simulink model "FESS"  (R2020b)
settings: Solver=VariableStepAuto  StartTime=0.0  StopTime=30  RelTol=1e-3
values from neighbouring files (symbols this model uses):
  C = 0    [FESS.m]
  F = 1    [FESS.m]
  f_el = 50    [FESS.m]
  P_load = 1500    [FESS.m]
  t_step = 5    [FESS.m]
undefined symbols (not defined in the file or in its folder): DCmot, DG
libraries: pid_lib x4, simulink x2

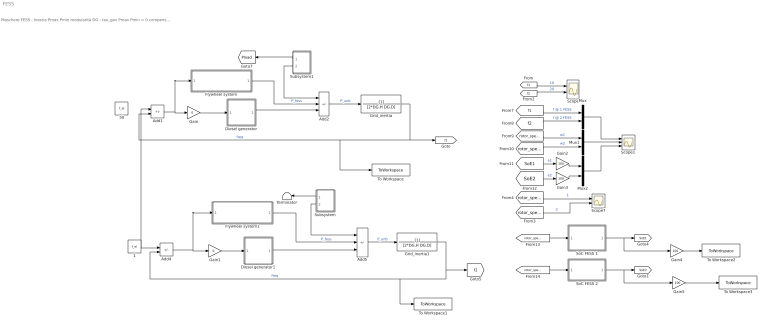
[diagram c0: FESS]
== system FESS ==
  note: Maschere FESS : Inerzia Pmax Pmin modularità DG : tau_gov Pmax Pmin = 0 compensazione FESS [0-1] Load : impulsi [0-1] step [0-1] Pstep Ptrain t/duty pulses
  1 : Constant  Value=f_el
  50 : Constant  Value=f_el
  Add1 : Sum  Inputs=+-
  Add2 : Sum  Inputs=-++
  Add4 : Sum  Inputs=+-
  Add5 : Sum  Inputs=-++
  Diesel generator : Subsystem  mask{s=[DG.tau_gov 1], W=4e5, O=-0.5, Gain=0}
      mask prompts: s "Tau_DG"; W "Upper limit P"; O "Lower limit P"; Gain "compensation"
  Diesel generator1 : Subsystem  mask{s=[DG.tau_gov 1], W=4e5, O=-0.5, Gain=0}
      mask prompts: s "Tau_DG"; W "Upper limit P"; O "Lower limit P"; Gain "compensation"
  Flywheel system : Subsystem  mask{J=20, Plim=DCmot.Pmax, Plim_neg=-DCmot.Pmax, Gain=1}
      mask prompts: J "Inerzia [kg*m^2]"; Plim "power limitation pos"; Plim_neg "power limitation neg"; Gain "Mod"
  Flywheel system1 : Subsystem  mask{J=20, Gain=1}
      mask prompts: J "Inerzia [kg*m^2]"; Gain "Mod"
  Gain : Gain  Gain=0
  Gain1 : Gain  Gain=0
  Gain{2..5} (4 alike) : Gain  Gain=100
  Grid_inertia : TransferFcn  Denominator=[2*DG.H DG.D]
  Grid_inertia1 : TransferFcn  Denominator=[2*DG.H DG.D]
  Mux : Mux  Inputs=2
  Mux1 : Mux  Inputs=2
  Mux2 : Mux  Inputs=2
  Scope : Scope  NumInputPorts=2
  Scope1 : Scope  NumInputPorts=3
  Scope7 : Scope  NumInputPorts=2
  SoC FESS 1 : Subsystem
  SoC FESS 2 : Subsystem
  Subsystem : Subsystem  mask{Gain=0, G=1, After=P_load, Amplitude=P_load, Period=3, PulseWidth=50}
      mask prompts: Gain "train"; G "step"; After "Pstep"; Amplitude "Puls amp"; Period "pulse durat"; PulseWidth "duty cycle"
  Subsystem1 : Subsystem  mask{Gain=1, G=0, After=P_load, Amplitude=P_load*2, Period=3, PulseWidth=50}
      mask prompts: Gain "train"; G "step"; After "Pstep"; Amplitude "Puls amp"; Period "pulse durat"; PulseWidth "duty cycle"
  Terminator : Terminator
  To Workspace : ToWorkspace  VariableName=f1  SaveFormat=Timeseries  SampleTime=-1
  To Workspace1 : ToWorkspace  VariableName=f2  SaveFormat=Timeseries  SampleTime=-1
  To Workspace2 : ToWorkspace  VariableName=Soe1  SaveFormat=Timeseries  SampleTime=-1
  To Workspace3 : ToWorkspace  VariableName=Soe2  SaveFormat=Timeseries  SampleTime=-1
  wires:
  Add1/1 -> Flywheel system/1(e_f), Gain/1
  Add2/1 -> Grid_inertia/1  "P_unb"
  50/1 -> Add1/1
  Grid_inertia/1 -> To Workspace/1, Add1/2, [f1]  "freq"
  Grid_inertia1/1 -> To Workspace1/1, Add4/2, [f2]  "freq"
  1/1 -> Add4/1
  Add5/1 -> Grid_inertia1/1  "P_unb"
  Add4/1 -> Flywheel system1/1(e_f), Gain1/1
  [f1] -> Scope/1  "10"
  Diesel generator/1(P_out) -> Add2/3
  Flywheel system1/1(P_FESS) -> Add5/2  "P_fess"
  Diesel generator1/1(P_out) -> Add5/3
  Subsystem/2(Pl) -> Add5/1
  Subsystem1/1(load) -> [Pload]
  Flywheel system/1(P_FESS) -> Add2/2  "P_fess"
  Subsystem1/2(Pl) -> Add2/1
  Subsystem/1(load) -> Terminator/1
  [f2] -> Scope/2  "20"
  Gain/1 -> Diesel generator/1(e_f)
  Gain1/1 -> Diesel generator1/1(e_f)
  [rotor_speed2] -> Scope7/2  "2"
  [rotor_speed2] -> SoC FESS 2/1(speed)
  SoC FESS 1/1(SoE) -> Gain4/1, [SoE1]
  [rotor_speed1] -> Scope7/1  "1"
  [rotor_speed1] -> SoC FESS 1/1(speed1)
  SoC FESS 2/1(SoE) -> Gain5/1, [SoE2]
  [rotor_speed1] -> Mux1/1  "w1"
  [SoE2] -> Gain3/1  "e2"
  [f1] -> Mux/1  "f @ 1 FESS"
  Mux/1 -> Scope1/1
  [f2] -> Mux/2  "f @ 2 FESS"
  [SoE1] -> Gain2/1  "e1"
  Mux1/1 -> Scope1/2
  [rotor_speed2] -> Mux1/2  "w2"
  Mux2/1 -> Scope1/3
  Gain2/1 -> Mux2/1
  Gain3/1 -> Mux2/2
  Gain4/1 -> To Workspace2/1
  Gain5/1 -> To Workspace3/1

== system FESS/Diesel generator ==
  note: aggiungo la Pload
  e_f : Inport
  Add : Sum
  Governor : TransferFcn  Denominator=s
  PI_DG : Subsystem
  Pload_compensation : Gain  Gain=Gain
  Saturation : Saturate  UpperLimit=W  LowerLimit=O
  P_out : Outport
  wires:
  Saturation/1 -> Governor/1
  Pload_compensation/1 -> Add/1
  Add/1 -> Saturation/1
  PI_DG/1(P_ref) -> Add/2
  e_f/1 -> PI_DG/1(e_f)
  [Pload] -> Pload_compensation/1
  Governor/1 -> P_out/1

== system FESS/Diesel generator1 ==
  note: aggiungo la Pload
  e_f : Inport
  Add : Sum
  Governor : TransferFcn  Denominator=s
  PI_DG : Subsystem
  Pload_compensation : Gain  Gain=Gain
  Saturation : Saturate  UpperLimit=W  LowerLimit=O
  P_out : Outport
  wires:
  Governor/1 -> P_out/1
  [Pload] -> Pload_compensation/1
  e_f/1 -> PI_DG/1(e_f)
  PI_DG/1(P_ref) -> Add/2
  Add/1 -> Saturation/1
  Pload_compensation/1 -> Add/1
  Saturation/1 -> Governor/1

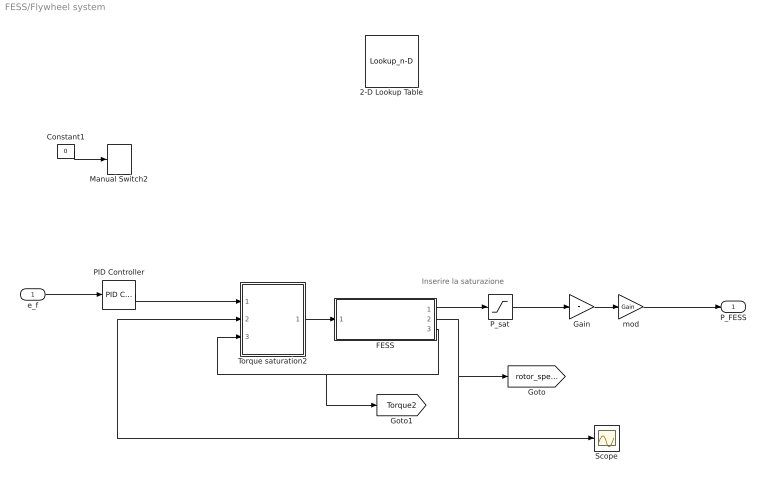
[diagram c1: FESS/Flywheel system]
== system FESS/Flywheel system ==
  note: Inserire la saturazione
  e_f : Inport
  2-D Lookup Table : Lookup_n-D  Commented=on  BreakpointsForDimension1=[1:3]  BreakpointsForDimension2=[1:3]  InternalRulePriority=Speed  RndMeth=Simplest
  Constant1 : Constant  Commented=on  Value=0
  FESS : Subsystem
  Gain : Gain  Gain=F
  Manual Switch2 : ManualSwitch  Commented=on  CurrentSetting=0
  PID Controller : pid_lib/PID Controller  Controller=PID  Form=Parallel  TimeDomain=Continuous-time  UseExternalTs=off  SampleTime=-1  IntegratorMethod=Forward Euler  FilterMethod=Forward Euler  ControllerParametersSource=internal  P=50*DCmot.Kt  I=100  D=0  UseFilter=on  N=100  TunerSelectOption=Transfer Function Based (PID Tuner App)  InitialConditionSource=internal  InitialConditionForIntegrator=0  InitialConditionForFilter=0  DifferentiatorICPrevScaledInput=0  ExternalReset=none  TrackingMode=off  Kt=1  LimitOutput=off  SatLimitsSource=internal  UpperSaturationLimit=inf  LowerSaturationLimit=-inf  LinearizeAsGain=on  AntiWindupMode=none  Kb=1  POutMin=[]  POutMax=[]  IOutMin=[]  IOutMax=[]  DOutMin=[]  DOutMax=[]  NOutMin=[]  NOutMax=[]  SumOutMin=[]  SumOutMax=[]  SaturationOutMin=[]  SaturationOutMax=[]  PParamMin=[]  PParamMax=[]  IParamMin=[]  IParamMax=[]  DParamMin=[]  DParamMax=[]  NParamMin=[]  NParamMax=[]  KbParamMin=[]  KbParamMax=[]  KtParamMin=[]  KtParamMax=[]  KbOutMin=[]  KbOutMax=[]  KtOutMin=[]  KtOutMax=[]  IntegratorOutMin=[]  IntegratorOutMax=[]  FilterOutMin=[]  FilterOutMax=[]  SumI1OutMin=[]  SumI1OutMax=[]  SumI2OutMin=[]  SumI2OutMax=[]  SumI3OutMin=[]  SumI3OutMax=[]  SumI4OutMin=[]  SumI4OutMax=[]  SumDOutMin=[]  SumDOutMax=[]  DifferentiatorOutMin=[]  DifferentiatorOutMax=[]  FilterDiffOutCoefMin=[]  FilterDiffOutCoefMax=[]  ReciprocalOutMin=[]  ReciprocalOutMax=[]  SumDenOutMin=[]  SumDenOutMax=[]  SumNumOutMin=[]  SumNumOutMax=[]  DivideOutMin=[]  DivideOutMax=[]  UdiffTsProdOutMin=[]  UdiffTsProdOutMax=[]  NTsProdOutMin=[]  NTsProdOutMax=[]  UintegralTsProdOutMin=[]  UintegralTsProdOutMax=[]  UngainTsProdOutMin=[]  UngainTsProdOutMax=[]  IntegratorContinuousStateAttributes=''  IntegratorStateMustResolveToSignalObject=off  IntegratorRTWStateStorageClass=Auto  FilterContinuousStateAttributes=''  FilterStateMustResolveToSignalObject=off  FilterRTWStateStorageClass=Auto  ParallelPVariant=InternalParameters  IdealPVariant=Disabled  IVariant=InternalParameters  DVariant=InternalParameters  IntegratorVariant=Continuous  SatVariant=Disabled  AWVariant=Passthrough  PCopyVariant=Disabled  TRVariant=Disabled  FdbkBlocksVariant=Forward  IdealPFdbkVariant=Disabled  SatFdbkVariant=Disabled  DerivativeFilterVariant=ContFilter  NVariant=InternalParameters  NCopyVariant=Disabled  FilterICVariant=InternalICsFilter  IntegratorICVariant=InternalICs  ExternalResetVariant=Disabled  TRSumVariant=Passthrough  SumFdbkVariant=Disabled  SumVariant=Sum_PID  TsampFilterVariant=InternalTs  TsampNgainVariant=Passthrough  TsampIntegralVariant=Passthrough  ExternalSaturationOutDataTypeStr=Inherit: Same as second input
  P_sat : Saturate  UpperLimit=Plim  LowerLimit=Plim_neg
  Scope : Scope
  Torque saturation2 : Subsystem
  mod : Gain  Gain=Gain
  P_FESS : Outport
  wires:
  e_f/1 -> PID Controller/1
  Torque saturation2/1(ia*) -> FESS/1(ia_ref)
  PID Controller/1 -> Torque saturation2/1(T*)
  FESS/2(w_r) -> [rotor_speed1], Torque saturation2/2(speed), Scope/1
  FESS/3(Tm) -> [Torque2], Torque saturation2/3(Torque)
  Constant1/1 -> Manual Switch2/1
  FESS/1(P_FESS) -> P_sat/1
  Gain/1 -> mod/1
  mod/1 -> P_FESS/1
  P_sat/1 -> Gain/1

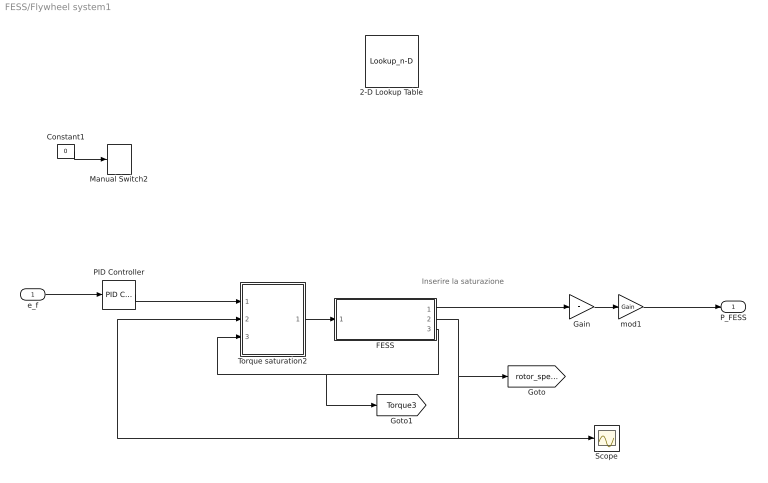
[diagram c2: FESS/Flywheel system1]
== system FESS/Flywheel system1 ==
  note: Inserire la saturazione
  e_f : Inport
  2-D Lookup Table : Lookup_n-D  Commented=on  BreakpointsForDimension1=[1:3]  BreakpointsForDimension2=[1:3]  InternalRulePriority=Speed  RndMeth=Simplest
  Constant1 : Constant  Commented=on  Value=0
  FESS : Subsystem
  Gain : Gain  Gain=F
  Manual Switch2 : ManualSwitch  Commented=on  CurrentSetting=0
  PID Controller : pid_lib/PID Controller  Controller=PID  Form=Parallel  TimeDomain=Continuous-time  UseExternalTs=off  SampleTime=-1  IntegratorMethod=Forward Euler  FilterMethod=Forward Euler  ControllerParametersSource=internal  P=50*DCmot.Kt  I=100  D=0  UseFilter=on  N=100  TunerSelectOption=Transfer Function Based (PID Tuner App)  InitialConditionSource=internal  InitialConditionForIntegrator=0  InitialConditionForFilter=0  DifferentiatorICPrevScaledInput=0  ExternalReset=none  TrackingMode=off  Kt=1  LimitOutput=off  SatLimitsSource=internal  UpperSaturationLimit=inf  LowerSaturationLimit=-inf  LinearizeAsGain=on  AntiWindupMode=none  Kb=1  POutMin=[]  POutMax=[]  IOutMin=[]  IOutMax=[]  DOutMin=[]  DOutMax=[]  NOutMin=[]  NOutMax=[]  SumOutMin=[]  SumOutMax=[]  SaturationOutMin=[]  SaturationOutMax=[]  PParamMin=[]  PParamMax=[]  IParamMin=[]  IParamMax=[]  DParamMin=[]  DParamMax=[]  NParamMin=[]  NParamMax=[]  KbParamMin=[]  KbParamMax=[]  KtParamMin=[]  KtParamMax=[]  KbOutMin=[]  KbOutMax=[]  KtOutMin=[]  KtOutMax=[]  IntegratorOutMin=[]  IntegratorOutMax=[]  FilterOutMin=[]  FilterOutMax=[]  SumI1OutMin=[]  SumI1OutMax=[]  SumI2OutMin=[]  SumI2OutMax=[]  SumI3OutMin=[]  SumI3OutMax=[]  SumI4OutMin=[]  SumI4OutMax=[]  SumDOutMin=[]  SumDOutMax=[]  DifferentiatorOutMin=[]  DifferentiatorOutMax=[]  FilterDiffOutCoefMin=[]  FilterDiffOutCoefMax=[]  ReciprocalOutMin=[]  ReciprocalOutMax=[]  SumDenOutMin=[]  SumDenOutMax=[]  SumNumOutMin=[]  SumNumOutMax=[]  DivideOutMin=[]  DivideOutMax=[]  UdiffTsProdOutMin=[]  UdiffTsProdOutMax=[]  NTsProdOutMin=[]  NTsProdOutMax=[]  UintegralTsProdOutMin=[]  UintegralTsProdOutMax=[]  UngainTsProdOutMin=[]  UngainTsProdOutMax=[]  IntegratorContinuousStateAttributes=''  IntegratorStateMustResolveToSignalObject=off  IntegratorRTWStateStorageClass=Auto  FilterContinuousStateAttributes=''  FilterStateMustResolveToSignalObject=off  FilterRTWStateStorageClass=Auto  ParallelPVariant=InternalParameters  IdealPVariant=Disabled  IVariant=InternalParameters  DVariant=InternalParameters  IntegratorVariant=Continuous  SatVariant=Disabled  AWVariant=Passthrough  PCopyVariant=Disabled  TRVariant=Disabled  FdbkBlocksVariant=Forward  IdealPFdbkVariant=Disabled  SatFdbkVariant=Disabled  DerivativeFilterVariant=ContFilter  NVariant=InternalParameters  NCopyVariant=Disabled  FilterICVariant=InternalICsFilter  IntegratorICVariant=InternalICs  ExternalResetVariant=Disabled  TRSumVariant=Passthrough  SumFdbkVariant=Disabled  SumVariant=Sum_PID  TsampFilterVariant=InternalTs  TsampNgainVariant=Passthrough  TsampIntegralVariant=Passthrough  ExternalSaturationOutDataTypeStr=Inherit: Same as second input
  Scope : Scope
  Torque saturation2 : Subsystem
  mod1 : Gain  Gain=Gain
  P_FESS : Outport
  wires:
  e_f/1 -> PID Controller/1
  Torque saturation2/1(ia*) -> FESS/1(ia_ref)
  PID Controller/1 -> Torque saturation2/1(T*)
  FESS/2(w_r) -> [rotor_speed2], Torque saturation2/2(speed), Scope/1
  FESS/3(Tm) -> [Torque3], Torque saturation2/3(Torque)
  Constant1/1 -> Manual Switch2/1
  FESS/1(P_FESS) -> Gain/1
  Gain/1 -> mod1/1
  mod1/1 -> P_FESS/1

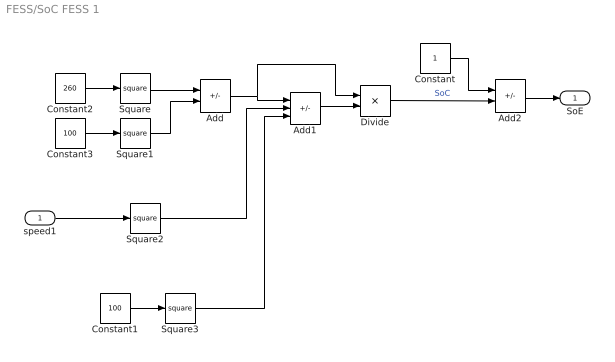
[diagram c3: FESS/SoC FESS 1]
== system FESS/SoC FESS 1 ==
  speed1 : Inport
  Add : Sum  Inputs=+-
  Add1 : Sum  Inputs=+-+
  Add2 : Sum  Inputs=+-
  Constant : Constant
  Constant1 : Constant  Value=100
  Constant2 : Constant  Value=260
  Constant3 : Constant  Value=100
  Divide : Product  Inputs=/*
  Square{,1..3} (4 alike) : Math  Operator=square
  SoE : Outport
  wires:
  Constant2/1 -> Square/1
  Divide/1 -> Add2/2  "SoC"
  Add1/1 -> Divide/2
  Add/1 -> Divide/1, Add1/1
  Constant3/1 -> Square1/1
  Square/1 -> Add/1
  Square1/1 -> Add/2
  Square2/1 -> Add1/2
  Square3/1 -> Add1/3
  Constant1/1 -> Square3/1
  Constant/1 -> Add2/1
  Add2/1 -> SoE/1
  speed1/1 -> Square2/1

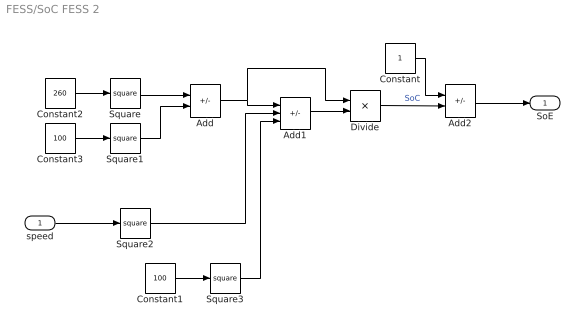
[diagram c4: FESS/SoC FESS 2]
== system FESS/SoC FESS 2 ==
  speed : Inport
  Add : Sum  Inputs=+-
  Add1 : Sum  Inputs=+-+
  Add2 : Sum  Inputs=+-
  Constant : Constant
  Constant1 : Constant  Value=100
  Constant2 : Constant  Value=260
  Constant3 : Constant  Value=100
  Divide : Product  Inputs=/*
  Square{,1..3} (4 alike) : Math  Operator=square
  SoE : Outport
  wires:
  Square2/1 -> Add1/2
  speed/1 -> Square2/1
  Square1/1 -> Add/2
  Square/1 -> Add/1
  Constant3/1 -> Square1/1
  Add/1 -> Add1/1, Divide/1
  Add1/1 -> Divide/2
  Divide/1 -> Add2/2  "SoC"
  Constant2/1 -> Square/1
  Constant1/1 -> Square3/1
  Square3/1 -> Add1/3
  Constant/1 -> Add2/1
  Add2/1 -> SoE/1

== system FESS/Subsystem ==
  Add : Sum
  P_load2 : Step  Time=t_step  After=After  SampleTime=0
  Positive Load1 : DiscretePulseGenerator  PulseType=Time based  Amplitude=Amplitude  Period=Period  PulseWidth=PulseWidth
  step : Gain  Gain=G
  train : Gain  Gain=Gain
  load : Outport
  Pl : Outport  Port=2
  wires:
  step/1 -> Add/1
  P_load2/1 -> step/1, load/1  "load"
  train/1 -> Add/2
  Positive Load1/1 -> train/1
  Add/1 -> Pl/1

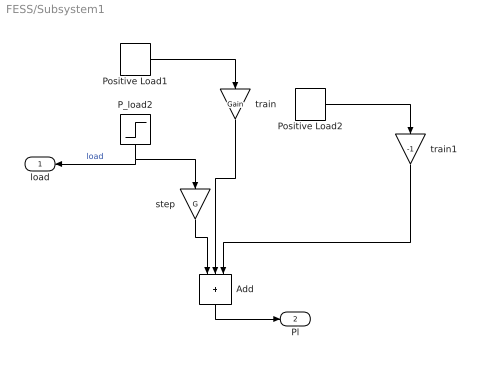
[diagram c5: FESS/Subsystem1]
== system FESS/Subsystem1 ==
  Add : Sum  Inputs=+++
  P_load2 : Step  Time=t_step  After=After  SampleTime=0
  Positive Load1 : DiscretePulseGenerator  PulseType=Time based  Amplitude=Amplitude  Period=Period  PulseWidth=PulseWidth
  Positive Load2 : DiscretePulseGenerator  PulseType=Time based  Amplitude=P_load  Period=3  PulseWidth=50  PhaseDelay=1.5
  step : Gain  Gain=G
  train : Gain  Gain=Gain
  train1 : Gain  Gain=-1
  load : Outport
  Pl : Outport  Port=2
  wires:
  step/1 -> Add/1
  P_load2/1 -> step/1, load/1  "load"
  train/1 -> Add/2
  Positive Load1/1 -> train/1
  Add/1 -> Pl/1
  Positive Load2/1 -> train1/1
  train1/1 -> Add/3

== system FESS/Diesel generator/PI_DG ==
  e_f : Inport
  Add : Sum
  Integrator : Integrator
  Ki,DG : Gain  Gain=DG.ki_dg
  Kp,DG : Gain  Gain=DG.kp_dg
  Manual Switch : ManualSwitch  CurrentSetting=0
  PID Controller : pid_lib/PID Controller  Controller=PID  Form=Parallel  TimeDomain=Continuous-time  UseExternalTs=off  SampleTime=-1  IntegratorMethod=Forward Euler  FilterMethod=Forward Euler  ControllerParametersSource=internal  P=DG.kp_dg  I=DG.ki_dg  D=0  UseFilter=on  N=100  TunerSelectOption=Transfer Function Based (PID Tuner App)  InitialConditionSource=internal  InitialConditionForIntegrator=0  InitialConditionForFilter=0  DifferentiatorICPrevScaledInput=0  ExternalReset=none  TrackingMode=off  Kt=1  LimitOutput=off  SatLimitsSource=internal  UpperSaturationLimit=inf  LowerSaturationLimit=-inf  LinearizeAsGain=on  AntiWindupMode=none  Kb=1  POutMin=[]  POutMax=[]  IOutMin=[]  IOutMax=[]  DOutMin=[]  DOutMax=[]  NOutMin=[]  NOutMax=[]  SumOutMin=[]  SumOutMax=[]  SaturationOutMin=[]  SaturationOutMax=[]  PParamMin=[]  PParamMax=[]  IParamMin=[]  IParamMax=[]  DParamMin=[]  DParamMax=[]  NParamMin=[]  NParamMax=[]  KbParamMin=[]  KbParamMax=[]  KtParamMin=[]  KtParamMax=[]  KbOutMin=[]  KbOutMax=[]  KtOutMin=[]  KtOutMax=[]  IntegratorOutMin=[]  IntegratorOutMax=[]  FilterOutMin=[]  FilterOutMax=[]  SumI1OutMin=[]  SumI1OutMax=[]  SumI2OutMin=[]  SumI2OutMax=[]  SumI3OutMin=[]  SumI3OutMax=[]  SumI4OutMin=[]  SumI4OutMax=[]  SumDOutMin=[]  SumDOutMax=[]  DifferentiatorOutMin=[]  DifferentiatorOutMax=[]  FilterDiffOutCoefMin=[]  FilterDiffOutCoefMax=[]  ReciprocalOutMin=[]  ReciprocalOutMax=[]  SumDenOutMin=[]  SumDenOutMax=[]  SumNumOutMin=[]  SumNumOutMax=[]  DivideOutMin=[]  DivideOutMax=[]  UdiffTsProdOutMin=[]  UdiffTsProdOutMax=[]  NTsProdOutMin=[]  NTsProdOutMax=[]  UintegralTsProdOutMin=[]  UintegralTsProdOutMax=[]  UngainTsProdOutMin=[]  UngainTsProdOutMax=[]  IntegratorContinuousStateAttributes=''  IntegratorStateMustResolveToSignalObject=off  IntegratorRTWStateStorageClass=Auto  FilterContinuousStateAttributes=''  FilterStateMustResolveToSignalObject=off  FilterRTWStateStorageClass=Auto  ParallelPVariant=InternalParameters  IdealPVariant=Disabled  IVariant=InternalParameters  DVariant=InternalParameters  IntegratorVariant=Continuous  SatVariant=Disabled  AWVariant=Passthrough  PCopyVariant=Disabled  TRVariant=Disabled  FdbkBlocksVariant=Forward  IdealPFdbkVariant=Disabled  SatFdbkVariant=Disabled  DerivativeFilterVariant=ContFilter  NVariant=InternalParameters  NCopyVariant=Disabled  FilterICVariant=InternalICsFilter  IntegratorICVariant=InternalICs  ExternalResetVariant=Disabled  TRSumVariant=Passthrough  SumFdbkVariant=Disabled  SumVariant=Sum_PID  TsampFilterVariant=InternalTs  TsampNgainVariant=Passthrough  TsampIntegralVariant=Passthrough  ExternalSaturationOutDataTypeStr=Inherit: Same as second input
  P_ref : Outport
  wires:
  Integrator/1 -> Add/2
  e_f/1 -> PID Controller/1, Ki,DG/1, Kp,DG/1
  Kp,DG/1 -> Add/1
  Ki,DG/1 -> Integrator/1
  Add/1 -> Manual Switch/2
  Manual Switch/1 -> P_ref/1
  PID Controller/1 -> Manual Switch/1

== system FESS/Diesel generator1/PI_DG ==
  e_f : Inport
  Add : Sum
  Integrator : Integrator
  Ki,DG : Gain  Gain=DG.ki_dg
  Kp,DG : Gain  Gain=DG.kp_dg
  Manual Switch : ManualSwitch  CurrentSetting=0
  PID Controller : pid_lib/PID Controller  Controller=PID  Form=Parallel  TimeDomain=Continuous-time  UseExternalTs=off  SampleTime=-1  IntegratorMethod=Forward Euler  FilterMethod=Forward Euler  ControllerParametersSource=internal  P=DG.kp_dg  I=DG.ki_dg  D=0  UseFilter=on  N=100  TunerSelectOption=Transfer Function Based (PID Tuner App)  InitialConditionSource=internal  InitialConditionForIntegrator=0  InitialConditionForFilter=0  DifferentiatorICPrevScaledInput=0  ExternalReset=none  TrackingMode=off  Kt=1  LimitOutput=off  SatLimitsSource=internal  UpperSaturationLimit=inf  LowerSaturationLimit=-inf  LinearizeAsGain=on  AntiWindupMode=none  Kb=1  POutMin=[]  POutMax=[]  IOutMin=[]  IOutMax=[]  DOutMin=[]  DOutMax=[]  NOutMin=[]  NOutMax=[]  SumOutMin=[]  SumOutMax=[]  SaturationOutMin=[]  SaturationOutMax=[]  PParamMin=[]  PParamMax=[]  IParamMin=[]  IParamMax=[]  DParamMin=[]  DParamMax=[]  NParamMin=[]  NParamMax=[]  KbParamMin=[]  KbParamMax=[]  KtParamMin=[]  KtParamMax=[]  KbOutMin=[]  KbOutMax=[]  KtOutMin=[]  KtOutMax=[]  IntegratorOutMin=[]  IntegratorOutMax=[]  FilterOutMin=[]  FilterOutMax=[]  SumI1OutMin=[]  SumI1OutMax=[]  SumI2OutMin=[]  SumI2OutMax=[]  SumI3OutMin=[]  SumI3OutMax=[]  SumI4OutMin=[]  SumI4OutMax=[]  SumDOutMin=[]  SumDOutMax=[]  DifferentiatorOutMin=[]  DifferentiatorOutMax=[]  FilterDiffOutCoefMin=[]  FilterDiffOutCoefMax=[]  ReciprocalOutMin=[]  ReciprocalOutMax=[]  SumDenOutMin=[]  SumDenOutMax=[]  SumNumOutMin=[]  SumNumOutMax=[]  DivideOutMin=[]  DivideOutMax=[]  UdiffTsProdOutMin=[]  UdiffTsProdOutMax=[]  NTsProdOutMin=[]  NTsProdOutMax=[]  UintegralTsProdOutMin=[]  UintegralTsProdOutMax=[]  UngainTsProdOutMin=[]  UngainTsProdOutMax=[]  IntegratorContinuousStateAttributes=''  IntegratorStateMustResolveToSignalObject=off  IntegratorRTWStateStorageClass=Auto  FilterContinuousStateAttributes=''  FilterStateMustResolveToSignalObject=off  FilterRTWStateStorageClass=Auto  ParallelPVariant=InternalParameters  IdealPVariant=Disabled  IVariant=InternalParameters  DVariant=InternalParameters  IntegratorVariant=Continuous  SatVariant=Disabled  AWVariant=Passthrough  PCopyVariant=Disabled  TRVariant=Disabled  FdbkBlocksVariant=Forward  IdealPFdbkVariant=Disabled  SatFdbkVariant=Disabled  DerivativeFilterVariant=ContFilter  NVariant=InternalParameters  NCopyVariant=Disabled  FilterICVariant=InternalICsFilter  IntegratorICVariant=InternalICs  ExternalResetVariant=Disabled  TRSumVariant=Passthrough  SumFdbkVariant=Disabled  SumVariant=Sum_PID  TsampFilterVariant=InternalTs  TsampNgainVariant=Passthrough  TsampIntegralVariant=Passthrough  ExternalSaturationOutDataTypeStr=Inherit: Same as second input
  P_ref : Outport
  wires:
  PID Controller/1 -> Manual Switch/1
  Manual Switch/1 -> P_ref/1
  Add/1 -> Manual Switch/2
  Ki,DG/1 -> Integrator/1
  Kp,DG/1 -> Add/1
  e_f/1 -> Kp,DG/1, Ki,DG/1, PID Controller/1
  Integrator/1 -> Add/2

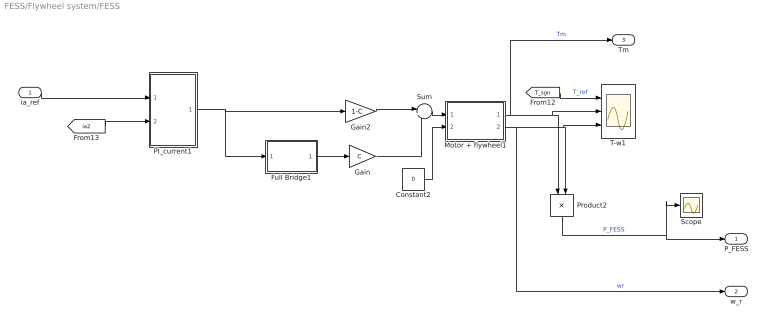
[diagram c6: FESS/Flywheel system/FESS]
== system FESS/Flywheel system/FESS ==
  ia_ref : Inport
  Constant2 : Constant  Value=0
  Full Bridge1 : Subsystem
  Gain : Gain  Gain=C
  Gain2 : Gain  Gain=1-C
  Motor + flywheel1 : Subsystem
  PI_current1 : Subsystem
  Product2 : Product
  Scope : Scope
  Sum : Sum  Inputs=|++
  T-w1 : Scope  NumInputPorts=3
  P_FESS : Outport
  w_r : Outport  Port=2
  Tm : Outport  Port=3
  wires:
  Motor + flywheel1/1(Tm) -> Tm/1, T-w1/2, Product2/1  "Tm"
  [ia2] -> PI_current1/2(ia_fbk)
  PI_current1/1(Va*) -> Gain2/1, Full Bridge1/1(Va_Ref)
  Constant2/1 -> Motor + flywheel1/2(Tr)
  Motor + flywheel1/2(wr) -> w_r/1, T-w1/3, Product2/2  "wr"
  [T_sgn] -> T-w1/1  "T_ref"
  ia_ref/1 -> PI_current1/1(ia*)
  Product2/1 -> Scope/1, P_FESS/1  "P_FESS"
  Full Bridge1/1(Va) -> Gain/1
  Gain2/1 -> Sum/1
  Sum/1 -> Motor + flywheel1/1(Va)
  Gain/1 -> Sum/2

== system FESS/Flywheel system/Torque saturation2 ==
  T* : Inport
  speed : Inport  Port=2
  Torque : Inport  Port=3
  Gain1 : Gain  Gain=1/DCmot.Kt
  Lookup with Linear Point-slope Interpolation : Lookup_n-D  NumberOfTableDimensions=1  BreakpointsForDimension1=[0,50,100,150,160,170,180,200,220,240,260]  Table=[0,0,0,1,1,1,1,1,1,1,0]  InternalRulePriority=Speed  RndMeth=Simplest
  MATLAB Function : MATLAB Function  Commented=on  TreatAsAtomicUnit=on
  Product2 : Product
  ia* : Outport
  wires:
  Lookup with Linear Point-slope Interpolation/1 -> Product2/2
  speed/1 -> Lookup with Linear Point-slope Interpolation/1
  Product2/1 -> Gain1/1
  T*/1 -> Product2/1
  Gain1/1 -> ia*/1
  Torque/1 -> MATLAB Function/2(T)

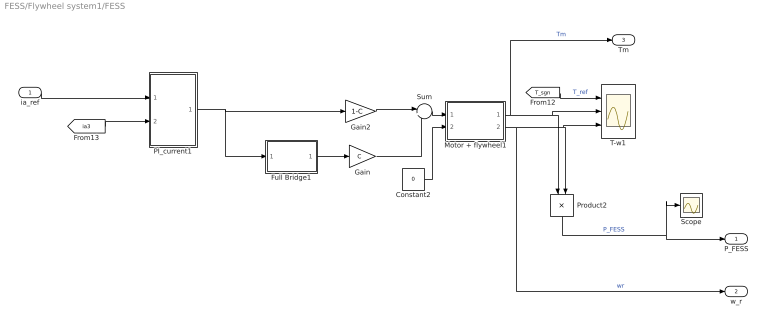
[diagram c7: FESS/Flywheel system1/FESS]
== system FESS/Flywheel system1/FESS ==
  ia_ref : Inport
  Constant2 : Constant  Value=0
  Full Bridge1 : Subsystem
  Gain : Gain  Gain=C
  Gain2 : Gain  Gain=1-C
  Motor + flywheel1 : Subsystem
  PI_current1 : Subsystem
  Product2 : Product
  Scope : Scope
  Sum : Sum  Inputs=|++
  T-w1 : Scope  NumInputPorts=3
  P_FESS : Outport
  w_r : Outport  Port=2
  Tm : Outport  Port=3
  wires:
  Motor + flywheel1/1(Tm) -> Tm/1, T-w1/2, Product2/1  "Tm"
  [ia3] -> PI_current1/2(ia_fbk)
  PI_current1/1(Va*) -> Gain2/1, Full Bridge1/1(Va_Ref)
  Constant2/1 -> Motor + flywheel1/2(Tr)
  Motor + flywheel1/2(wr) -> w_r/1, T-w1/3, Product2/2  "wr"
  [T_sgn] -> T-w1/1  "T_ref"
  ia_ref/1 -> PI_current1/1(ia*)
  Product2/1 -> Scope/1, P_FESS/1  "P_FESS"
  Full Bridge1/1(Va) -> Gain/1
  Gain2/1 -> Sum/1
  Sum/1 -> Motor + flywheel1/1(Va)
  Gain/1 -> Sum/2

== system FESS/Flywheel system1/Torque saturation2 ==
  T* : Inport
  speed : Inport  Port=2
  Torque : Inport  Port=3
  Gain1 : Gain  Gain=1/DCmot.Kt
  Lookup with Linear Point-slope Interpolation : Lookup_n-D  NumberOfTableDimensions=1  BreakpointsForDimension1=[0,50,100,150,160,170,180,200,220,240,260]  Table=[0,0,0,1,1,1,1,1,1,1,0]  InternalRulePriority=Speed  RndMeth=Simplest
  MATLAB Function : MATLAB Function  Commented=on  TreatAsAtomicUnit=on
  Product2 : Product
  ia* : Outport
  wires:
  Lookup with Linear Point-slope Interpolation/1 -> Product2/2
  speed/1 -> Lookup with Linear Point-slope Interpolation/1
  Product2/1 -> Gain1/1
  T*/1 -> Product2/1
  Gain1/1 -> ia*/1
  Torque/1 -> MATLAB Function/2(T)

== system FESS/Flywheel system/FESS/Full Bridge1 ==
  Va_Ref : Inport
  Converter : Subsystem
  Unipolar PWM : Subsystem
  Va : Outport  VectorParamsAs1DForOutWhenUnconnected=off
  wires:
  Va_Ref/1 -> Unipolar PWM/1(Va_Rref)
  Unipolar PWM/1(dA) -> Converter/1(dA)
  Unipolar PWM/2(dB) -> Converter/2(dB)
  Converter/1(Va) -> Va/1

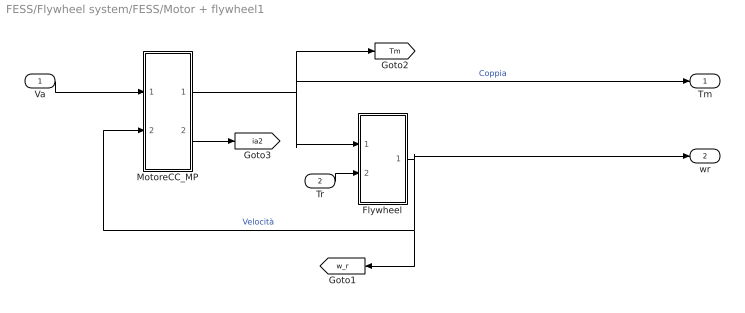
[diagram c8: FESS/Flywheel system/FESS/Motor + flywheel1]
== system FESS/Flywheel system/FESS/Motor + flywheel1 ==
  Va : Inport
  Tr : Inport  Port=2
  Flywheel : Subsystem
  MotoreCC_MP : Subsystem
  Tm : Outport
  wr : Outport  Port=2
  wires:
  Va/1 -> MotoreCC_MP/1(Va)
  Tr/1 -> Flywheel/2(Cr)
  MotoreCC_MP/1(Cm) -> Tm/1, Flywheel/1(Cm), [Tm]  "Coppia"
  MotoreCC_MP/2(ia) -> [ia2]
  Flywheel/1(wr) -> wr/1, [w_r], MotoreCC_MP/2(wr)  "Velocità"

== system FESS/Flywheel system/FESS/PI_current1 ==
  ia* : Inport
  ia_fbk : Inport  Port=2
  Add : Sum  Inputs=+-
  current PI : Subsystem
  Va* : Outport
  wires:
  current PI/1(Va*) -> Va*/1
  ia_fbk/1 -> Add/2
  ia*/1 -> Add/1
  Add/1 -> current PI/1(e_i)

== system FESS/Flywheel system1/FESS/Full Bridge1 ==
  Va_Ref : Inport
  Converter : Subsystem
  Unipolar PWM : Subsystem
  Va : Outport  VectorParamsAs1DForOutWhenUnconnected=off
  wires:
  Va_Ref/1 -> Unipolar PWM/1(Va_Rref)
  Unipolar PWM/1(dA) -> Converter/1(dA)
  Unipolar PWM/2(dB) -> Converter/2(dB)
  Converter/1(Va) -> Va/1

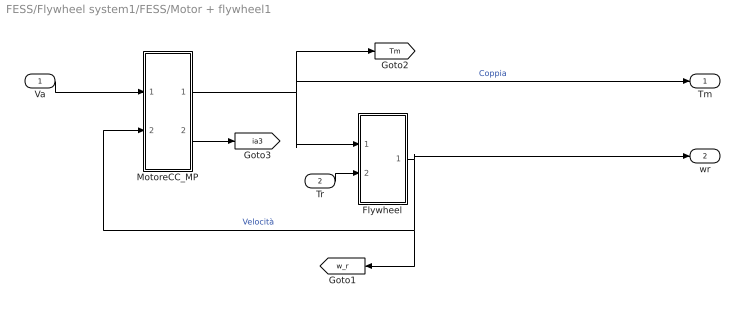
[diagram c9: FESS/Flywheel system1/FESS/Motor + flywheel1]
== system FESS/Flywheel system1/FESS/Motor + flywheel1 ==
  Va : Inport
  Tr : Inport  Port=2
  Flywheel : Subsystem
  MotoreCC_MP : Subsystem
  Tm : Outport
  wr : Outport  Port=2
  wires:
  Va/1 -> MotoreCC_MP/1(Va)
  Tr/1 -> Flywheel/2(Cr)
  MotoreCC_MP/1(Cm) -> Tm/1, Flywheel/1(Cm), [Tm]  "Coppia"
  MotoreCC_MP/2(ia) -> [ia3]
  Flywheel/1(wr) -> wr/1, [w_r], MotoreCC_MP/2(wr)  "Velocità"

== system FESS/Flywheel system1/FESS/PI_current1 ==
  ia* : Inport
  ia_fbk : Inport  Port=2
  Add : Sum  Inputs=+-
  current PI : Subsystem
  Va* : Outport
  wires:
  current PI/1(Va*) -> Va*/1
  ia_fbk/1 -> Add/2
  ia*/1 -> Add/1
  Add/1 -> current PI/1(e_i)

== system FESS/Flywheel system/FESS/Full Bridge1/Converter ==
  dA : Inport
  dB : Inport  Port=2
  Gain : Gain  Gain=DCmot.Van
  Sum : Sum  Inputs=+|-
  Va : Outport  VectorParamsAs1DForOutWhenUnconnected=off
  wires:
  Sum/1 -> Gain/1
  Gain/1 -> Va/1
  dB/1 -> Sum/2
  dA/1 -> Sum/1

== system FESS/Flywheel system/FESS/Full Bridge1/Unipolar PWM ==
  Va_Rref : Inport
  Fcn : Fcn  Expr=0.5*(1 + u(1)/DCmot.Van) > u(2)
  Fcn1 : Fcn  Expr=0.5*(1 - u(1)/DCmot.Van) > u(2)
  Mux : Mux  Inputs=2
  Repeating Sequence : simulink/Sources/Repeating Sequence  rep_seq_t=DCmot.Tsw*[0 0.5 1]  rep_seq_y=[1 0 1]
  dA : Outport  VectorParamsAs1DForOutWhenUnconnected=off
  dB : Outport  Port=2  VectorParamsAs1DForOutWhenUnconnected=off
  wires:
  Fcn1/1 -> dB/1
  Fcn/1 -> dA/1
  Repeating Sequence/1 -> Mux/2
  Mux/1 -> Fcn/1, Fcn1/1
  Va_Rref/1 -> Mux/1

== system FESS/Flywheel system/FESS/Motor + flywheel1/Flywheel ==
  note: Coppia ventilante
  Cm : Inport
  Cr : Inport  Port=2
  Divide : Product  Inputs=*/
  Gain1 : Gain  Gain=0
  Inertia_1 : Constant  Value=J
  Integrator : Integrator  InitialCondition=120
  Subtract : Sum  Inputs=---
  wr : Outport
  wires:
  Gain1/1 -> Subtract/1
  Cm/1 -> Subtract/2
  Cr/1 -> Subtract/3
  Integrator/1 -> wr/1, Gain1/1
  Subtract/1 -> Divide/1
  Divide/1 -> Integrator/1
  Inertia_1/1 -> Divide/2

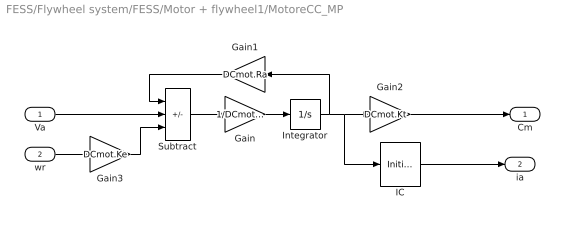
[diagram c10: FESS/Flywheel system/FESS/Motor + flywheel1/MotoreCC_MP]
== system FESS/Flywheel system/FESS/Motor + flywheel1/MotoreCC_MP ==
  Va : Inport
  wr : Inport  Port=2
  Gain : Gain  Gain=1/DCmot.La
  Gain1 : Gain  Gain=DCmot.Ra
  Gain2 : Gain  Gain=DCmot.Kt
  Gain3 : Gain  Gain=DCmot.Ke
  IC : InitialCondition  Value=DCmot.I_reg
  Integrator : Integrator
  Subtract : Sum  Inputs=-+-
  Cm : Outport
  ia : Outport  Port=2
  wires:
  IC/1 -> ia/1
  Gain2/1 -> Cm/1
  Gain1/1 -> Subtract/1
  Va/1 -> Subtract/2
  Integrator/1 -> Gain1/1, IC/1, Gain2/1
  Subtract/1 -> Gain/1
  Gain/1 -> Integrator/1
  Gain3/1 -> Subtract/3
  wr/1 -> Gain3/1

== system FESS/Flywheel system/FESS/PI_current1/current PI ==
  e_i : Inport
  Add : Sum
  Gain : Gain  Gain=DCmot.kii
  Gain1 : Gain  Gain=DCmot.kpi
  Integrator : Integrator
  anti wind-up : Saturate  UpperLimit=DCmot.I_reg  LowerLimit=-DCmot.I_reg
  Va* : Outport
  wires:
  Integrator/1 -> anti wind-up/1
  Gain/1 -> Integrator/1
  Gain1/1 -> Add/1
  anti wind-up/1 -> Add/2
  e_i/1 -> Gain/1, Gain1/1
  Add/1 -> Va*/1

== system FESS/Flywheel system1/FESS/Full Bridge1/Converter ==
  dA : Inport
  dB : Inport  Port=2
  Gain : Gain  Gain=DCmot.Van
  Sum : Sum  Inputs=+|-
  Va : Outport  VectorParamsAs1DForOutWhenUnconnected=off
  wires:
  Sum/1 -> Gain/1
  Gain/1 -> Va/1
  dB/1 -> Sum/2
  dA/1 -> Sum/1

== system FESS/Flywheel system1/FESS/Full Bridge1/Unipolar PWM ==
  Va_Rref : Inport
  Fcn : Fcn  Expr=0.5*(1 + u(1)/DCmot.Van) > u(2)
  Fcn1 : Fcn  Expr=0.5*(1 - u(1)/DCmot.Van) > u(2)
  Mux : Mux  Inputs=2
  Repeating Sequence : simulink/Sources/Repeating Sequence  rep_seq_t=DCmot.Tsw*[0 0.5 1]  rep_seq_y=[1 0 1]
  dA : Outport  VectorParamsAs1DForOutWhenUnconnected=off
  dB : Outport  Port=2  VectorParamsAs1DForOutWhenUnconnected=off
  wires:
  Fcn1/1 -> dB/1
  Fcn/1 -> dA/1
  Repeating Sequence/1 -> Mux/2
  Mux/1 -> Fcn/1, Fcn1/1
  Va_Rref/1 -> Mux/1

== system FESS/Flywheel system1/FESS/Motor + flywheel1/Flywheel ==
  note: Coppia ventilante
  Cm : Inport
  Cr : Inport  Port=2
  Divide : Product  Inputs=*/
  Gain1 : Gain  Gain=0
  Inertia_1 : Constant  Value=J
  Integrator : Integrator  InitialCondition=120
  Subtract : Sum  Inputs=---
  wr : Outport
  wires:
  Gain1/1 -> Subtract/1
  Cm/1 -> Subtract/2
  Cr/1 -> Subtract/3
  Integrator/1 -> wr/1, Gain1/1
  Subtract/1 -> Divide/1
  Divide/1 -> Integrator/1
  Inertia_1/1 -> Divide/2

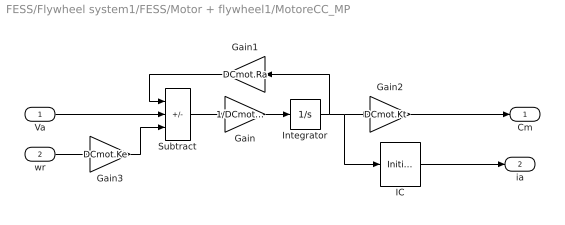
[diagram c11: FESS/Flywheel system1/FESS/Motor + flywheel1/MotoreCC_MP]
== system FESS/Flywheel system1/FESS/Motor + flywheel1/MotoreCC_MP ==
  Va : Inport
  wr : Inport  Port=2
  Gain : Gain  Gain=1/DCmot.La
  Gain1 : Gain  Gain=DCmot.Ra
  Gain2 : Gain  Gain=DCmot.Kt
  Gain3 : Gain  Gain=DCmot.Ke
  IC : InitialCondition  Value=DCmot.I_reg
  Integrator : Integrator
  Subtract : Sum  Inputs=-+-
  Cm : Outport
  ia : Outport  Port=2
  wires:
  IC/1 -> ia/1
  Gain2/1 -> Cm/1
  Gain1/1 -> Subtract/1
  Va/1 -> Subtract/2
  Integrator/1 -> Gain1/1, IC/1, Gain2/1
  Subtract/1 -> Gain/1
  Gain/1 -> Integrator/1
  Gain3/1 -> Subtract/3
  wr/1 -> Gain3/1

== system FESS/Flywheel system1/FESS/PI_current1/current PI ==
  e_i : Inport
  Add : Sum
  Gain : Gain  Gain=DCmot.kii
  Gain1 : Gain  Gain=DCmot.kpi
  Integrator : Integrator
  anti wind-up : Saturate  UpperLimit=DCmot.I_reg  LowerLimit=-DCmot.I_reg
  Va* : Outport
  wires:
  Integrator/1 -> anti wind-up/1
  Gain/1 -> Integrator/1
  Gain1/1 -> Add/1
  anti wind-up/1 -> Add/2
  e_i/1 -> Gain/1, Gain1/1
  Add/1 -> Va*/1

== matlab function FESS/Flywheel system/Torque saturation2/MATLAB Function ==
function out = fcn(u,T)
%La convenzione è quella degli utilizzatori: T positiva -> Motore
%                                            T negativa -> Generatore  
y = 0; %inizializzazione uscita

if (u>100 && u<250)     % qualsiasi sia il segno della coppia, questa viene fornita
    y=1;
elseif (u>250 && T<0)   % la velocità è alta ma il FESS sta generando
    y=1;                % viene fornita Coppia
    
elseif (u>250 && T>0)   % Il volano non può più accumulare energia (limite Motore)
    y=0;                % non viene fornite Coppia
    
elseif (u<100 && T<0)   % Il volano ha ceduto tutta l'energia accumulata (limite Generatore)
    y=0;                % non viene fornite Coppia
    
elseif (u<100 && T>0)   % la valocità è bassa ma il FESS sta accumulando
    y=1;                % viene fornita Coppia
    
elseif T*u > 140e3      % saturazione di potenza
    y=0;                % non viene fornita coppia 
end

out = y;

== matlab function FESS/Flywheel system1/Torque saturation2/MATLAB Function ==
function out = fcn(u,T)
%La convenzione è quella degli utilizzatori: T positiva -> Motore
%                                            T negativa -> Generatore  
y = 0; %inizializzazione uscita

if (u>100 && u<250)     % qualsiasi sia il segno della coppia, questa viene fornita
    y=1;
elseif (u>250 && T<0)   % la velocità è alta ma il FESS sta generando
    y=1;                % viene fornita Coppia
    
elseif (u>250 && T>0)   % Il volano non può più accumulare energia (limite Motore)
    y=0;                % non viene fornite Coppia
    
elseif (u<100 && T<0)   % Il volano ha ceduto tutta l'energia accumulata (limite Generatore)
    y=0;                % non viene fornite Coppia
    
elseif (u<100 && T>0)   % la valocità è bassa ma il FESS sta accumulando
    y=1;                % viene fornita Coppia
    
elseif T*u > 140e3      % saturazione di potenza
    y=0;                % non viene fornita coppia 
end

out = y;
